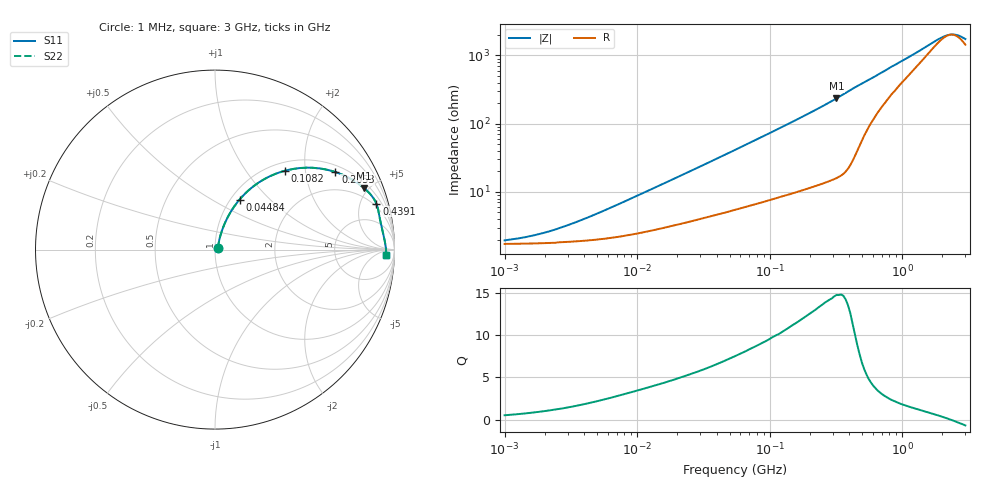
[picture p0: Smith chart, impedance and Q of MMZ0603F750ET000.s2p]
! S-Parameter Data Generated by TDK Corporation
! Copyright(C) 2025 TDK Corporation.
! All Rights Reserved.
! TDK P/N: MMZ0603F750ET000 (Chip Bead)
! Property: |Z|=75ohm at 100MHz
! Size(LxWxT): 0.6x0.3x0.3mm
! Model Type: s2p (Touchstone File Format Version 1.0)
! Frequency: DC=Yes Start=1MHz Stop=3000MHz 202points Log-sweep
! Model Generated on Feb. 6, 2025
! Terms and conditions regarding TDK Simulation Models:
! 1)This simulation model is being provided solely for informational
!  purposes. Please refer to the specifications of the products in
!  terms of detailed characteristics of such products.
! 2)In no event shall TDK Corporation of any of its subsidiaries be
!  liable for any loss or damage arising, directly or indirectly,
!  from any information contained in this simulation model, including,
!  but not limited to loss or damages arising from any inaccuracies,
!  omissions or errors in connection with such information.
! 3)Any and all copyrights on this simulation model are owned by
!  TDK Corporation.  Duplication or redistribution of this simulation
!  model without prior written permission from TDK Corporation
!  is prohibited.
! 4)This simulation model is subject to any modification or change
!  without any prior notice.
! 5)Neither TDK Corporation nor any of its subsidiaries shall make any
!  warranty, express or implied, including but not limited to the
!  correctness, implied warranties of merchantability and fitness for
!  a particular purpose with respect to this simulation models.
! 6)The use of this simulation model shall be deemed to have consented
!  to the terms and conditions hereof.
! Port Assignments:
!  1 ---@@@--- 2
! Applicable Conditions:
!  Temperature = 25 degC
!  DC Bias Current = 0 A
!  Small Signal Operation
# Hz S MA R 50
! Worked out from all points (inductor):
!   201 points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, 1 MHz to 3 GHz, reference 50 ohm
!   read as one part in series: L = 134 nH near 8.018 MHz
!   highest Q = 14.7 at 318.8 MHz (marker M1), where L = 117 nH
!   self-resonance near 2.326 GHz
!   S11 on the Smith chart (normalised r, x): 1 MHz: 1.03, +0.02; 44.84 MHz: 1.10, +0.68; 108.2 MHz: 1.16, +1.56; 205.3 MHz: 1.23, +2.93; 439.1 MHz: 1.67, +6.76; 3 GHz: 30, -20
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1000000  0.01915 27.0  0.983 -0.5  0.983 -0.5  0.01915 27.0
1433740  0.02133 35.8  0.9828 -0.7  0.9828 -0.7  0.02133 35.8
1897447  0.02413 43.0  0.9825 -1.0  0.9825 -1.0  0.02413 43.0
2412589  0.02759 49.1  0.9821 -1.2  0.9821 -1.2  0.02759 49.1
3900413  0.03869 59.0  0.9807 -1.9  0.9807 -1.9  0.03869 59.0
8017732  0.07043 67.9  0.9757 -3.8  0.9757 -3.8  0.07043 67.9
1.461624e7  0.119 69.9  0.9656 -6.6  0.9656 -6.6  0.119 69.9
2.773354e7  0.2073 68.1  0.9426 -11.8  0.9426 -11.8  0.2073 68.1
4.483659e7  0.3104 63.9  0.9071 -17.9  0.9071 -17.9  0.3104 63.9
5.477226e7  0.3645 61.2  0.8844 -21.2  0.8844 -21.2  0.3645 61.2
7.544761e7  0.4639 55.9  0.8336 -27.4  0.8336 -27.4  0.4639 55.9
1.081723e8  0.5887 48.4  0.7511 -35.9  0.7511 -35.9  0.5887 48.4
1.49005e8  0.6997 40.7  0.6549 -44.2  0.6549 -44.2  0.6997 40.7
2.052512e8  0.7979 32.8  0.5432 -52.7  0.5432 -52.7  0.7979 32.8
2.136344e8  0.8087 31.8  0.5286 -53.7  0.5286 -53.7  0.8087 31.8
3.188066e8  0.898 22.5  0.3833 -63.6  0.3833 -63.6  0.898 22.5
4.391493e8  0.9348 15.9  0.2751 -68.5  0.2751 -68.5  0.9348 15.9
8.005644e8  0.9375 7.6  0.1431 -60.4  0.1431 -60.4  0.9375 7.6
2.092429e9  0.9518 0.7  0.04961 -13.3  0.04961 -13.3  0.9518 0.7
2.455801e9  0.9534 -0.4  0.04706 7.5  0.04706 7.5  0.9534 -0.4
2.660507e9  0.9538 -0.9  0.04867 18.1  0.04867 18.1  0.9538 -0.9
3e9  0.9542 -1.8  0.05486 32.6  0.05486 32.6  0.9542 -1.8
